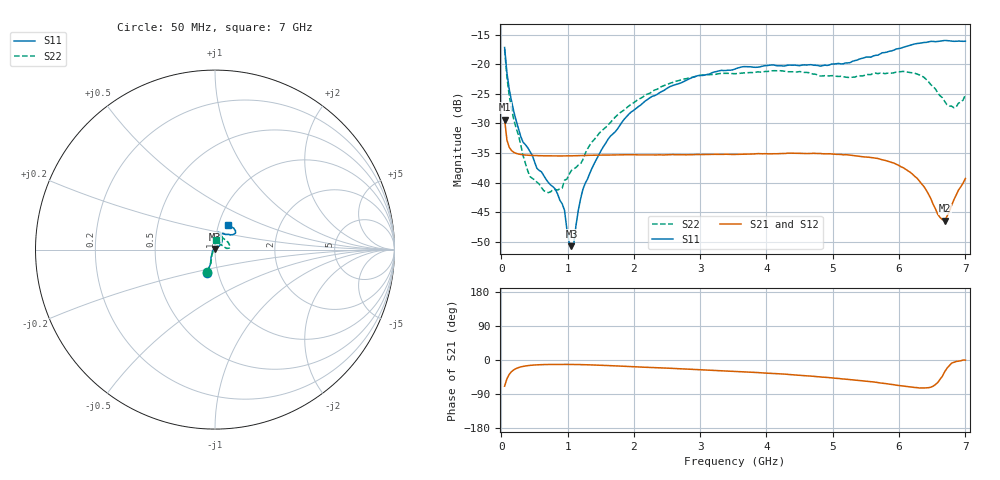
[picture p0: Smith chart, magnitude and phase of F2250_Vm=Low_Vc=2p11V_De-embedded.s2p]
! Integrated Device Technology
! Corporate Headquarters
! 6024 Silver Creek Valley Road
! San Jose, CA 95138  USA
! Phone:  1-408-284-8200
! Toll Free:  1-800-223-1366
! Webpage:  http://www.idt.com/
! Timing and RF Division
! 515 Groton Road, Suite 102
! Westford, MA 01886-6024
! Device:  F2250
! Description: Voltage Variable RF Attenuator
! Frequency:  50.0 -  6000.00 MHz
! Package:  3x3 mm Thin QFN Plastic Package: 16 pin
! Ports:  2 RF, 3 DC
!  Pin  1  = GND
!  Pin  2  = NC
!  Pin  3  = RF1  = Port 1
!  Pin  4  = NC
!  Pin  5  = GND
!  Pin  6  = GND
!  Pin  7  = GND
!  Pin  8  = GND
!  Pin  9  = NC
!  Pin 10  = RF2  = Port 2
!  Pin 11  = NC
!  Pin 12  = GND
!  Pin 13  = GND
!  Pin 14  = VCNTRL
!  Pin 15  = VDD
!  Pin 16  = VMODE
! Vcntrl:  2.110 Volts
! Vmode:  +0.000 Volts
! Vdd:  +3.30  Volts
! Current:  1.179 mA
! Data:  The device was measured on a the F2250 evaluation board which has
!  individual transmission lines to the RF pins.  Data was collected
!  using a calibrated network analyzer.  The evaluation board was
!  de-embedded using a TRL calibration technique.
!  The reference plane is the edge of the package pin.
! Misc:  SN 10
!  Action Tracker AT0258
! Date Measured:  2014-11-26
! Date:  2015-10-15  MJV
! Note:
!  Integrated Device Technology supplies this data as a sample of measured
!  data at the package pin for this product.  Your particular data for this
!  product may vary.
!  Data was taken at 25 degrees C.
!  Integrated Device Technology reserves the right to change this data at anytime.
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# GHz S dB R 50
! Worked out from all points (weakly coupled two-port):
!   201 points, 50 MHz to 7 GHz, reference 50 ohm
!   highest |S21| = -29.35 dB at 50 MHz (marker M1); lowest = -46.4 dB at 6.687 GHz (marker M2)
!   lowest |S11| = -50.7 dB at 1.058 GHz (marker M3), VSWR 1.01, Z = 49.8 + j0.243 ohm
!   |S11| at or under -10 dB: start of sweep to end of sweep
!   |S22| runs from -41.7 to -17.5 dB; largest |S21 - S12| = 5.7e-05
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0.05  -17.18 -108.6  -29.35 -69.1  -29.35 -69.0  -17.54 -109.8
0.08475  -21.44 -107.4  -32.79 -49.7  -32.79 -49.7  -22.12 -107.2
0.189  -28.00 -119.7  -34.88 -25.9  -34.87 -25.9  -29.37 -119.8
0.328  -33.16 -133.8  -35.30 -16.8  -35.30 -16.8  -35.43 -134.1
0.43225  -34.73 -144.6  -35.39 -14.2  -35.39 -14.2  -38.97 -160.3
0.6755  -39.44 -163.7  -35.48 -11.9  -35.47 -11.9  -41.56 152.3
0.91875  -43.58 158.1  -35.49 -11.6  -35.49 -11.6  -40.92 113.9
0.9535  -44.67 169.9  -35.49 -11.6  -35.49 -11.6  -39.59 113.7
1.023  -50.08 143.7  -35.48 -11.7  -35.48 -11.7  -38.60 95.0
1.05775  -50.73 122.9  -35.47 -11.7  -35.47 -11.7  -37.93 90.1
1.0925  -50.39 89.3  -35.46 -11.8  -35.47 -11.8  -37.71 85.2
1.162  -44.67 56.7  -35.45 -12.0  -35.45 -12.0  -37.03 74.2
1.2315  -41.10 44.2  -35.42 -12.3  -35.42 -12.2  -36.11 65.7
1.6485  -32.12 42.0  -35.33 -14.9  -35.34 -14.9  -29.81 54.7
2.37825  -24.88 47.3  -35.30 -20.6  -35.30 -20.6  -24.07 51.8
3.525  -20.80 72.5  -35.23 -30.0  -35.23 -30.0  -21.60 72.3
4.7065  -20.17 72.3  -35.05 -43.1  -35.05 -43.1  -21.66 70.9
5.85325  -17.82 40.5  -36.46 -63.7  -36.46 -63.7  -21.47 20.4
6.33975  -16.40 41.0  -40.20 -73.7  -40.22 -73.8  -21.97 6.2
6.68725  -15.99 48.8  -46.44 -31.2  -46.44 -30.7  -26.28 26.3
6.82625  -16.14 53.6  -42.90 -6.1  -42.86 -6.0  -27.35 52.8
7  -16.12 63.3  -39.31 -0.2  -39.28 -0.4  -25.16 85.1
